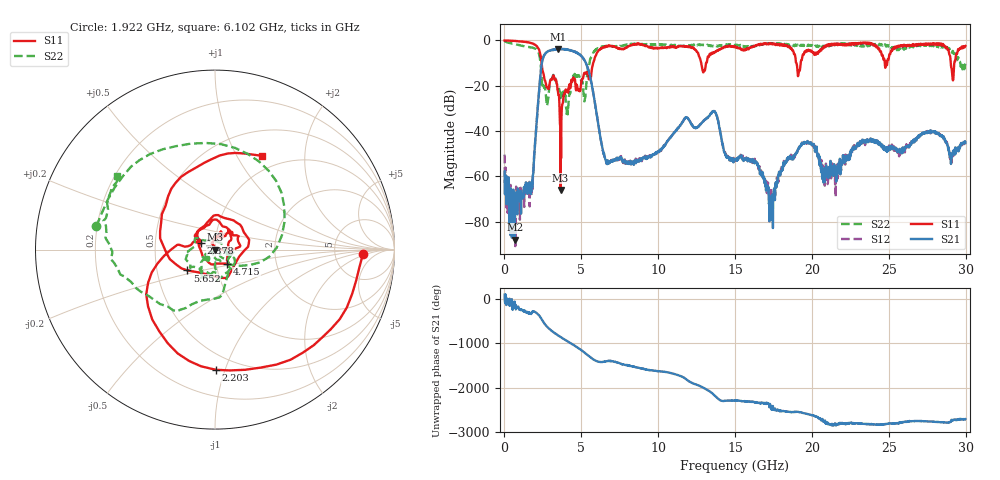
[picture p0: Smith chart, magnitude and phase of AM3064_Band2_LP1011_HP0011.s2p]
# Hz S DB R 50.0
!freq dBS11 angS11 dBS21 angS21 dBS12 angS12 dBS22 angS22
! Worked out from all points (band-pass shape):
!   1600 points, 10 MHz to 29.98 GHz, reference 50 ohm
!   highest |S21| = -3.73 dB at 3.515 GHz (marker M1); lowest = -88.0 dB at 666 MHz (marker M2)
!   |S21| within 3 dB of the highest: 2.571 GHz to 4.979 GHz (2.407 GHz wide, 63.8 % of centre)
!   lowest |S11| = -66.0 dB at 3.646 GHz (marker M3), VSWR 1.00, Z = 50 + j0.024 ohm
!   |S11| at or under -10 dB: 2.414 GHz to 5.772 GHz (3.358 GHz wide, 82 % of centre); 12.8 GHz to 13.11 GHz (313.1 MHz wide, 2.42 % of centre); 18.99 GHz to 19.27 GHz (279.4 MHz wide, 1.46 % of centre)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
!   |S22| runs from -33.5 to -0.3 dB; largest |S21 - S12| = 0.023
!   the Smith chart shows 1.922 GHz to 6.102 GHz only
!   S11 on the Smith chart (normalised r, x): 1.922 GHz: 10, -2; 2.203 GHz: 0.38, -0.93; 2.878 GHz: 0.85, +0.07; 4.715 GHz: 1.13, -0.18; 5.652 GHz: 0.72, -0.17; 6.102 GHz: 0.81, +1.28
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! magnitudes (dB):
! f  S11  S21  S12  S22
! 10 MHz  0.0  -57.9  -50.4  -0.3
! 666 MHz  -0.3  -88.0  -74.6  -1.6
! 1.922 GHz  -1.7  -52.8  -51.5  -3.4
! 2.203 GHz  -3.5  -26.4  -26.4  -5.2
! 2.878 GHz  -21.2  -4.6  -4.6  -23.5
! 3.515 GHz  -24.1  -3.7  -3.9  -22.3
! 3.646 GHz  -66.0  -3.9  -3.8  -25.5
! 4.715 GHz  -19.8  -5.6  -5.4  -15.3
! 5.015 GHz  -17.5  -7.0  -7.0  -18.5
! 5.652 GHz  -14.3  -18.6  -18.5  -7.3
! 6.102 GHz  -4.7  -36.8  -36.8  -3.3
! 6.72 GHz  -2.5  -53.0  -54.7  -2.4
! 10 GHz  -3.4  -49.0  -49.4  -1.9
! 13.6 GHz  -5.4  -31.5  -31.3  -2.6
! 15 GHz  -2.7  -52.7  -53.1  -1.9
! 16.39 GHz  -2.1  -54.1  -54.1  -2.3
! 17.35 GHz  -1.4  -69.8  -71.4  -1.2
! 18.27 GHz  -2.3  -53.3  -52.7  -1.9
! 19.99 GHz  -4.8  -46.1  -45.6  -2.1
! 20.93 GHz  -2.2  -55.2  -58.9  -2.2
! 25 GHz  -8.0  -47.1  -47.8  -2.2
! 29.98 GHz  -2.5  -45.4  -44.7  -10.3
